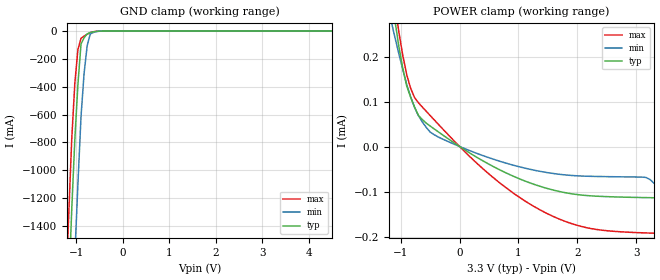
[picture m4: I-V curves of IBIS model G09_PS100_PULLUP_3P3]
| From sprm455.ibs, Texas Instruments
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|   Model Cell G09_PS100_PULLUP_3P3
|IDG09_PS100_PULLUP_3P3
[Model]   G09_PS100_PULLUP_3P3
Model_type   Input
Polarity   Non-Inverting
Vinl =  0.8V
Vinh =  2V
C_comp   1.447p   1.213p   1.874p
[Model Spec]
Vinl   0.8V   0.8V   0.8V
Vinh   2V   2V   2V
[Temperature Range]   25   125   -40
[Voltage Range]   3.3   3   3.6
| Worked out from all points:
|   GND clamp passes 1 mA (typ) near -0.53 V on its own axis
|   POWER clamp passes 1 mA (typ) near -1.78 V on its own axis
[POWER_clamp]
|   voltage   I(typ)   I(min)   I(max)
-3.3V     2.696mA    1.572mA    4.068mA
-1.167V   346.5uA    280.4uA    410.2uA
-1.1V     280.7uA    242.8uA    316.3uA
-1.033V   222.7uA    206.6uA    254.9uA
-900mV    135.1uA    138.3uA    160uA
-700mV    69.06uA    68.47uA    97.2uA
-500mV    45.48uA    32.08uA    68.8uA
33.33mV   -2.83uA    -1.789uA   -4.359uA
900mV     -65.25uA   -41.07uA   -102.3uA
1.633V    -98.05uA   -60.66uA   -157.8uA
2.3V      -110.2uA   -66.43uA   -183.8uA
3.3V      -113.8uA   -81.06uA   -192.6uA
[GND_clamp]
|   voltage   I(typ)   I(min)   I(max)
-3.3V     -22.54A    -23.36A    -22.09A
-1.233V   -2.454A    -3.359A    -1.924A
-1.167V   -1.863A    -2.762A    -1.341A
-1.1V     -1.287A    -2.174A    -780.3mA
-1.033V   -782.2mA   -1.619A    -375.6mA
-966.7mV  -384.2mA   -1.1A      -133mA
-900mV    -93.06mA   -616.1mA   -52.53mA
-833.3mV  -47.66mA   -302.3mA   -36.31mA
-766.7mV  -20.08mA   -103.8mA   -22.33mA
-700mV    -10.34mA   -20.43mA   -10.6mA
-366.7mV  -127uA     -153.7uA   -196.2uA
6.6V      0A         0A         0A
